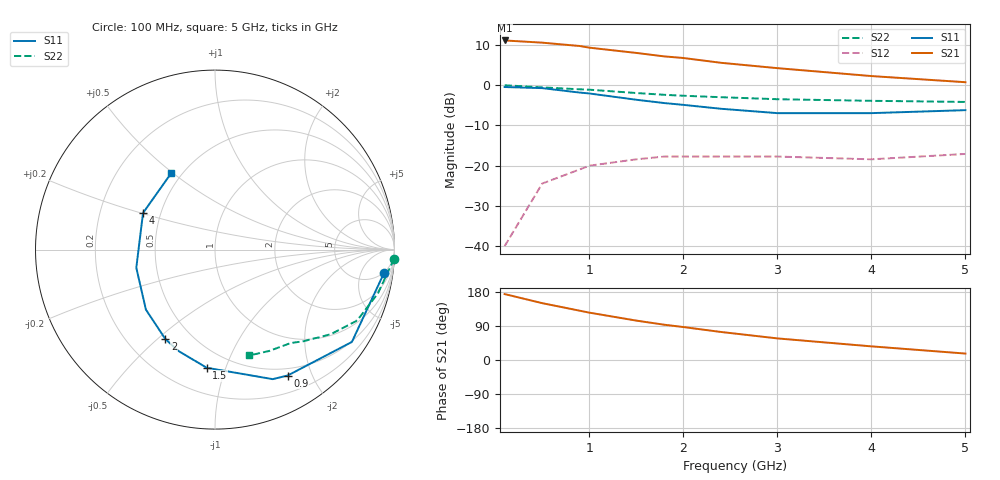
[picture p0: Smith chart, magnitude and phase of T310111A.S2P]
!AT-31011
!S and NOISE PARAMETERS at Vce=1V  Ic=1mA.  LAST UPDATED 06-23-94
# ghz s ma r 50
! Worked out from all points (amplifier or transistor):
!   11 points, 100 MHz to 5 GHz, reference 50 ohm
!   highest |S21| = 11.1 dB at 100 MHz (marker M1)
!   |S21| within 3 dB of that: start of sweep to 1.463 GHz
!   unconditionally stable (mu >= 1): 2.952 GHz to end of sweep
!   at 500 MHz: K = 0.19, MSG = 17.5 dB, |S12| = -24.4 dB
!   at 1.8 GHz: K = 0.58, MSG = 12.4 dB, |S12| = -17.7 dB
!   at 5 GHz: K = 1.31, MAG = 5.6 dB, |S12| = -17.1 dB
!   lowest NFmin = 0.50 dB at 500 MHz
!   S11 on the Smith chart (normalised r, x): 100 MHz: 5, -13; 900 MHz: 0.41, -1.66; 1.5 GHz: 0.37, -0.86; 2 GHz: 0.36, -0.53; 4 GHz: 0.40, +0.20; 5 GHz: 0.44, +0.49
0.1  0.95 -8.0  3.6 174.0  0.01 85.0  0.999 -3.0
0.5  0.92 -34.0  3.38 150.0  0.06 68.0  0.94 -15.0
0.9  0.81 -60.0  3.07 130.0  0.09 53.0  0.89 -25.0
1  0.79 -66.0  2.93 125.0  0.1 50.0  0.88 -27.0
1.5  0.66 -94.0  2.52 104.0  0.12 36.0  0.8 -36.0
1.8  0.6 -110.0  2.28 93.0  0.13 30.0  0.76 -40.0
2  0.57 -119.0  2.18 87.0  0.13 27.0  0.74 -42.0
2.4  0.51 -139.0  1.9 74.0  0.13 22.0  0.71 -46.0
3  0.45 -167.0  1.63 57.0  0.13 19.0  0.67 -51.0
4  0.45 153.0  1.3 36.0  0.12 22.0  0.64 -62.0
5  0.49 120.0  1.09 17.0  0.14 32.0  0.62 -72.0
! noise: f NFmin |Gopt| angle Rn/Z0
0.5  0.5  0.902  13  0.85
0.9  0.6  0.85  29  0.73
1.8  1.1  0.68  67  0.46
2.4  1.6  0.55  98  0.28
